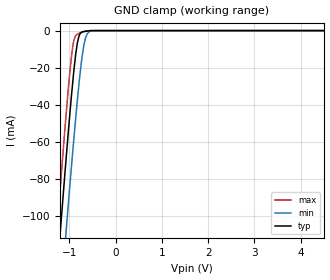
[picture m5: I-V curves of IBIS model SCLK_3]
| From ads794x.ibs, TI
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|   SCLK 3.3V Model
[Model] SCLK_3
Model_type   Input
Vinl = 0.99
Vinh = 2.31
|   typ   min   max
|   (Nom PVT)   (Fast PVT)  (Slow PVT)
C_comp   8.4973470e-13   7.0307390e-13   1.0010000e-12
|POWER = 3.3v
[Model Spec]
Vinl   0.99   0.9   1.08
Vinh   2.31   2.1   2.52
|Vinl = 0.3 X DVDD
|Vinh = 0.7 X DVDD
[Voltage Range]   3.3   3   3.6
[Temperature Range]   27   125   -40
[Power Clamp Reference]   3.3   3   3.6
[GND Clamp Reference]   0   0   0
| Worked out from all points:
|   GND clamp passes 1 mA (typ) near -0.74 V on its own axis
[GND Clamp]
|   Voltage   I(typ)   I(min)   I(max)
-3.3V     -821.8mA   -851.7mA   -804.8mA
-1.274V   -133.6mA   -172.6mA   -109.8mA
-1.191V   -106.6mA   -145.9mA   -82.69mA
-1.091V   -75.13mA   -114.5mA   -51.13mA
-1.035V   -58.06mA   -97.15mA   -34.43mA
-925mV    -27.16mA   -64.45mA   -8.184mA
-829.4mV  -6.955mA   -38.07mA   -2.026mA
-723.5mV  -668.5uA   -13.78mA   -835.8uA
-677.9mV  -498.6uA   -6.75mA    -472.6uA
-614.2mV  -260.7uA   -1.748mA   -217uA
-440.3mV  -20.36uA   -24.09uA   -20.25uA
6.59V     0A         0A         0A
[POWER Clamp]
|   SCR cell for ESD function. Effects occurr above VDD x 2
|   Voltage   I(typ)   I(min)   I(max)
-3.3V     0A         0A         0A
0V        0A         0A         0A
6.6V      0A         0A         0A
